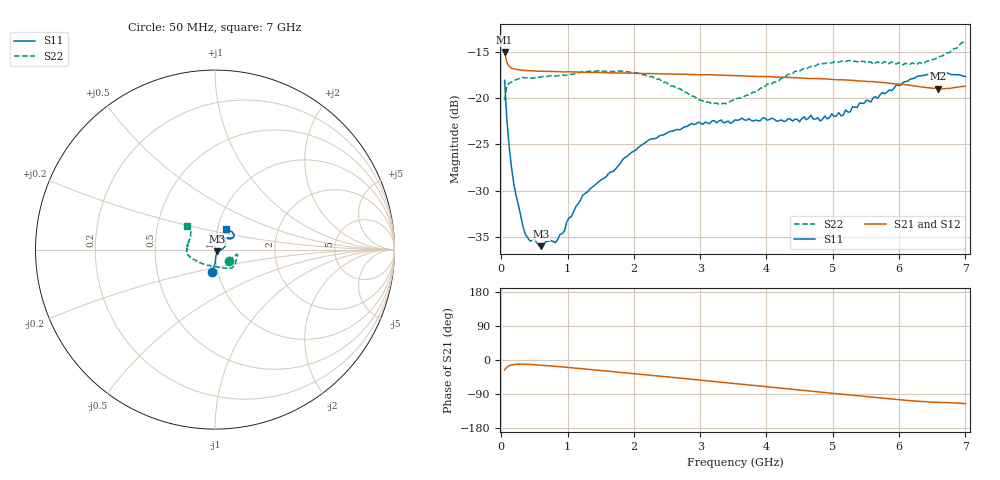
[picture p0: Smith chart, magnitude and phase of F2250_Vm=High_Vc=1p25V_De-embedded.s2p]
! Integrated Device Technology
! Corporate Headquarters
! 6024 Silver Creek Valley Road
! San Jose, CA 95138  USA
! Phone:  1-408-284-8200
! Toll Free:  1-800-223-1366
! Webpage:  http://www.idt.com/
! Timing and RF Division
! 515 Groton Road, Suite 102
! Westford, MA 01886-6024
! Device:  F2250
! Description: Voltage Variable RF Attenuator
! Frequency:  50.0 -  6000.00 MHz
! Package:  3x3 mm Thin QFN Plastic Package: 16 pin
! Ports:  2 RF, 3 DC
!  Pin  1  = GND
!  Pin  2  = NC
!  Pin  3  = RF1  = Port 1
!  Pin  4  = NC
!  Pin  5  = GND
!  Pin  6  = GND
!  Pin  7  = GND
!  Pin  8  = GND
!  Pin  9  = NC
!  Pin 10  = RF2  = Port 2
!  Pin 11  = NC
!  Pin 12  = GND
!  Pin 13  = GND
!  Pin 14  = VCNTRL
!  Pin 15  = VDD
!  Pin 16  = VMODE
! Vcntrl:  1.250 Volts
! Vmode:  +3.300 Volts
! Vdd:  +3.30  Volts
! Current:  1.333 mA
! Data:  The device was measured on a the F2250 evaluation board which has
!  individual transmission lines to the RF pins.  Data was collected
!  using a calibrated network analyzer.  The evaluation board was
!  de-embedded using a TRL calibration technique.
!  The reference plane is the edge of the package pin.
! Misc:  SN 10
!  Action Tracker AT0258
! Date Measured:  2014-11-26
! Date:  2015-10-15  MJV
! Note:
!  Integrated Device Technology supplies this data as a sample of measured
!  data at the package pin for this product.  Your particular data for this
!  product may vary.
!  Data was taken at 25 degrees C.
!  Integrated Device Technology reserves the right to change this data at anytime.
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# GHz S dB R 50
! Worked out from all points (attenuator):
!   201 points, 50 MHz to 7 GHz, reference 50 ohm
!   highest |S21| = -15.04 dB at 50 MHz (marker M1); lowest = -19.0 dB at 6.583 GHz (marker M2)
!   lowest |S11| = -36.0 dB at 606 MHz (marker M3), VSWR 1.03, Z = 51.4 - j0.862 ohm
!   |S11| at or under -10 dB: start of sweep to end of sweep
!   |S22| runs from -20.7 to -13.8 dB; largest |S21 - S12| = 0.0005
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0.05  -18.09 -97.2  -15.04 -26.1  -15.03 -26.0  -20.26 -39.2
0.08475  -22.40 -89.1  -16.19 -18.7  -16.18 -18.7  -18.68 -19.1
0.1195  -25.29 -86.7  -16.58 -15.0  -16.58 -15.0  -18.40 -13.8
0.189  -29.31 -79.8  -16.85 -11.9  -16.84 -11.9  -18.12 -12.0
0.22375  -30.60 -74.7  -16.90 -11.3  -16.90 -11.3  -18.02 -12.4
0.36275  -34.72 -58.1  -17.02 -11.2  -17.02 -11.2  -17.82 -13.3
0.606  -36.00 -32.0  -17.10 -13.7  -17.09 -13.7  -17.70 -19.7
0.8145  -35.62 -18.4  -17.15 -16.7  -17.13 -16.7  -17.64 -25.4
0.9535  -34.35 -21.6  -17.18 -18.8  -17.15 -18.8  -17.57 -29.3
0.98825  -33.37 -20.2  -17.16 -19.3  -17.15 -19.4  -17.52 -30.1
1.2315  -30.49 -8.3  -17.21 -23.2  -17.19 -23.3  -17.15 -35.6
1.96125  -25.89 12.8  -17.32 -35.3  -17.31 -35.3  -17.20 -48.4
2.37825  -24.12 23.6  -17.37 -42.3  -17.37 -42.4  -17.94 -56.9
3.07325  -22.62 45.3  -17.48 -54.3  -17.48 -54.3  -20.44 -86.5
3.525  -22.36 59.4  -17.58 -62.2  -17.58 -62.2  -20.21 -117.8
4.7065  -22.27 66.4  -17.89 -82.8  -17.88 -82.8  -16.59 -165.8
5.15825  -21.85 49.3  -18.04 -90.7  -18.05 -90.7  -16.00 -175.0
5.193  -21.30 49.5  -18.04 -91.3  -18.06 -91.3  -16.05 -175.9
5.85325  -19.12 34.9  -18.41 -102.5  -18.39 -102.7  -16.27 168.5
6.27025  -17.66 35.3  -18.73 -108.8  -18.73 -108.8  -16.34 155.2
6.583  -17.41 41.8  -18.99 -111.8  -19.00 -111.9  -15.62 144.4
7  -17.67 62.5  -18.72 -115.0  -18.73 -115.1  -13.78 139.8
